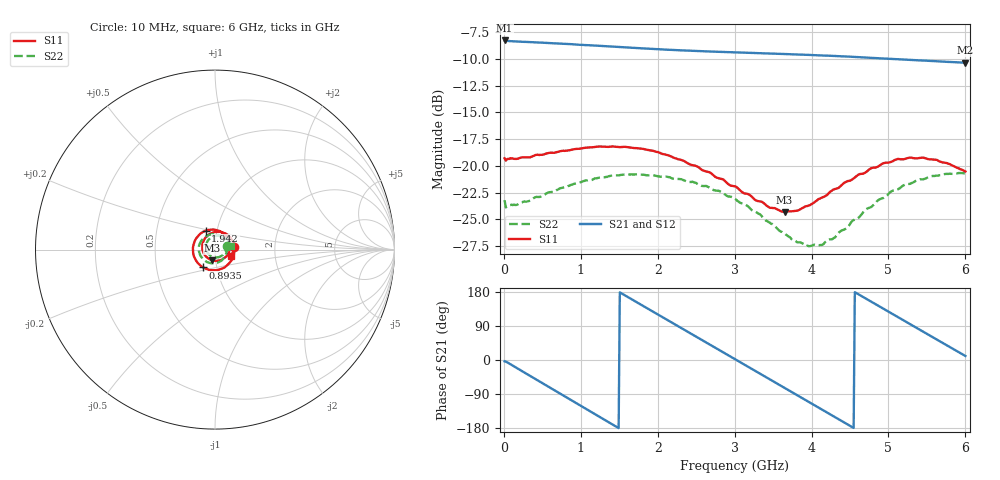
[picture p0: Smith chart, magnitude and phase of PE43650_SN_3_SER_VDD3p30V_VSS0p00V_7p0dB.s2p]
!Keysight Technologies,N5245B,MY57181451,A.13.50.07
!Date: Tuesday, May 07, 2019 07:59:58
!Correction: S11(Full 2 Port(1,2))
!S21(Full 2 Port(1,2))
!S12(Full 2 Port(1,2))
!S22(Full 2 Port(1,2))
!S2P File: Measurements: S11, S21, S12, S22:
# Hz S  dB  R 50
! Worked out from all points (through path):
!   401 points, 10 MHz to 6 GHz, reference 50 ohm
!   highest |S21| = -8.28 dB at 10 MHz (marker M1); lowest = -10.4 dB at 6 GHz (marker M2)
!   group delay of S21, straight-line fit = 327 ps
!   lowest |S11| = -24.3 dB at 3.649 GHz (marker M3), VSWR 1.13, Z = 48.1 - j5.67 ohm
!   |S11| at or under -10 dB: start of sweep to end of sweep
!   |S22| runs from -27.5 to -20.7 dB; largest |S21 - S12| = 0.0033
!   S11 on the Smith chart (normalised r, x): 10 MHz: 1.24, +0.04; 893.5 MHz: 0.86, -0.17; 1.942 GHz: 0.88, +0.19; 6 GHz: 1.19, -0.09
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1e7  -19.29 8.0  -8.28 -3.3  -8.35 -3.2  -23.19 17.2
2.496e8  -19.19 -36.6  -8.40 -30.9  -8.45 -30.9  -23.34 -35.7
5.04175e8  -18.95 -72.4  -8.48 -61.7  -8.54 -61.7  -22.80 -71.7
8.93525e8  -18.46 -123.4  -8.63 -108.5  -8.69 -108.5  -21.72 -120.2
1.013325e9  -18.36 -138.4  -8.69 -122.8  -8.74 -122.8  -21.47 -134.1
1.252925e9  -18.19 -166.7  -8.78 -151.3  -8.84 -151.3  -21.08 -159.7
1.47755e9  -18.22 167.4  -8.87 -178.0  -8.94 -177.9  -20.88 177.1
1.941775e9  -18.59 116.1  -9.07 127.2  -9.13 127.2  -20.87 132.0
2.01665e9  -18.75 108.2  -9.10 118.4  -9.15 118.5  -20.98 125.2
2.241275e9  -19.31 83.5  -9.18 92.0  -9.23 92.1  -21.23 103.8
2.4659e9  -19.94 58.2  -9.25 65.7  -9.30 65.7  -21.51 82.5
2.750425e9  -21.03 25.7  -9.33 32.3  -9.38 32.4  -22.30 54.4
3.005e9  -21.90 -6.9  -9.39 2.4  -9.44 2.5  -23.06 27.9
3.3045e9  -23.29 -49.6  -9.46 -32.8  -9.51 -32.7  -24.43 -8.0
3.648925e9  -24.30 -105.5  -9.55 -73.3  -9.60 -73.3  -26.30 -55.7
4.008325e9  -23.53 -165.5  -9.64 -115.7  -9.68 -115.6  -27.42 -117.6
4.277875e9  -22.22 154.9  -9.71 -147.5  -9.77 -147.4  -26.79 -164.7
4.517475e9  -21.31 122.9  -9.80 -175.7  -9.85 -175.6  -25.24 157.7
4.757075e9  -20.29 94.2  -9.89 156.0  -9.94 156.2  -23.89 127.8
5.01165e9  -19.67 66.8  -9.99 126.2  -10.04 126.4  -22.52 98.1
5.4609e9  -19.24 22.4  -10.16 73.5  -10.20 73.7  -21.23 55.2
6e9  -20.52 -23.4  -10.36 10.6  -10.41 10.7  -20.71 11.3
